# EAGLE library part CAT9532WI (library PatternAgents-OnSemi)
16-bit Programmable LED Dimmer with I2C Interface
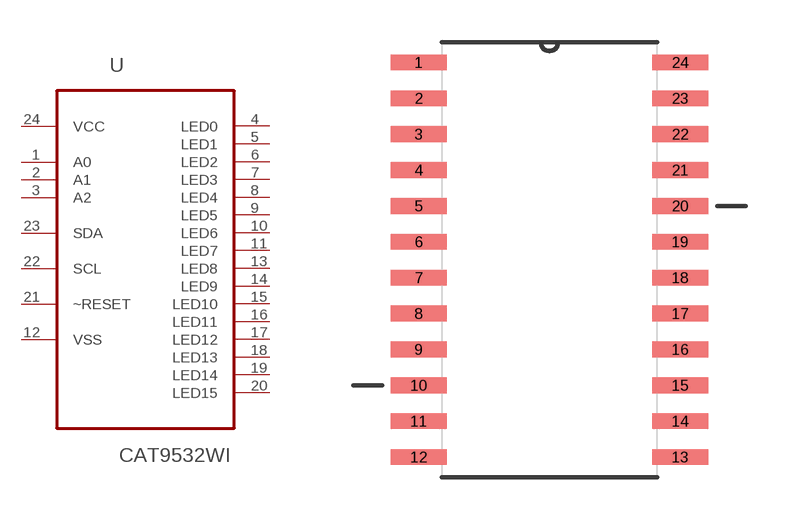
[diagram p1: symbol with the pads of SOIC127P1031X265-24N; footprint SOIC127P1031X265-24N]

Designator prefix U

## CAT9532WI (MPN: CAT9532WI.; OC_FARNELL: 1656134; OC_NEWARK: 11P0275; PACKAGE: SOIC-24; SUPPLIER: On Semiconductor)  [SOIC127P1031X265-24N]
1  A0  in
2  A1  in
3  A2  in
4  LED0  out
5  LED1  out
6  LED2  out
7  LED3  out
8  LED4  out
9  LED5  out
10  LED6  out
11  LED7  out
12  VSS  in
13  LED8  out
14  LED9  out
15  LED10  out
16  LED11  out
17  LED12  out
18  LED13  out
19  LED14  out
20  LED15  out
21  ~RESET  in
22  SCL  in
23  SDA  in
24  VCC  pwr

## Footprint SOIC127P1031X265-24N (pad centres in mm)
smd 1.981 x 0.559: 1 -4.623,6.985; 2 -4.623,5.715; 3 -4.623,4.445; 4 -4.623,3.175; 5 -4.623,1.905; 6 -4.623,0.635; 7 -4.623,-0.635; 8 -4.623,-1.905; 9 -4.623,-3.175; 10 -4.623,-4.445; 11 -4.623,-5.715; 12 -4.623,-6.985; 13 4.623,-6.985; 14 4.623,-5.715; 15 4.623,-4.445; 16 4.623,-3.175; 17 4.623,-1.905; 18 4.623,-0.635; 19 4.623,0.635; 20 4.623,1.905; 21 4.623,3.175; 22 4.623,4.445; 23 4.623,5.715; 24 4.623,6.985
